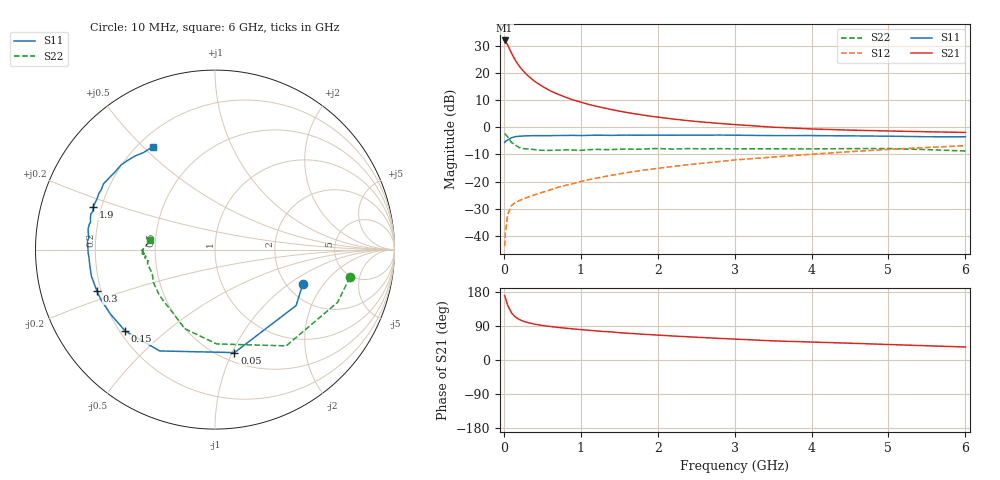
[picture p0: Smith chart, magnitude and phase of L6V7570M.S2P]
!  INFINEON TECHNOLOGIES Small Signal Semiconductors
! BFR380L3 , Si-NPN RF-Transistor in TSLP-3-1
!  Vce=0.75 V,  Ic=70 mA
! Common Emitter S-Parameters:  07. March 2005
#  GHz  S  MA  R  50
! f  S11  S21  S12  S22
! GHz  Mag  Ang  Mag  Ang  Mag  Ang  Mag  Ang
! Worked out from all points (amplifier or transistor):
!   36 points, 10 MHz to 6 GHz, reference 50 ohm
!   highest |S21| = 32.1 dB at 10 MHz (marker M1)
!   |S21| within 3 dB of that: start of sweep to 71.65 MHz
!   unconditionally stable (mu >= 1): 752.4 MHz to end of sweep
!   at 250 MHz: K = 0.60, MSG = 23.7 dB, |S12| = -26.4 dB
!   at 1.4 GHz: K = 1.11, MAG = 10.1 dB, |S12| = -17.7 dB
!   at 6 GHz: K = 1.04, MAG = 1.2 dB, |S12| = -6.8 dB
!   S11 on the Smith chart (normalised r, x): 10 MHz: 2.42, -1.30; 50 MHz: 0.59, -1.02; 150 MHz: 0.22, -0.37; 300 MHz: 0.18, -0.17; 1.9 GHz: 0.17, +0.17; 6 GHz: 0.26, +0.54
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0.01  0.5257 -21.7  40.24 170.2  0.0064 65.1  0.7671 -11.6
0.02  0.5491 -34.6  39.1 164.5  0.0113 69.1  0.7433 -23.3
0.05  0.584 -79.3  33.12 144.4  0.0247 56.1  0.6672 -53.5
0.1  0.6431 -118.6  23.39 124.2  0.036 44.5  0.5257 -89.0
0.15  0.6753 -137.8  17.24 113.3  0.0412 41.0  0.4717 -111.0
0.2  0.6842 -148.3  13.51 107.0  0.0444 41.3  0.424 -123.5
0.25  0.6933 -155.7  11.09 102.5  0.0476 41.1  0.4051 -135.2
0.3  0.6973 -160.5  9.319 99.3  0.0507 42.8  0.4004 -141.1
0.4  0.7043 -167.9  7.095 94.5  0.0567 46.3  0.3887 -152.1
0.5  0.7031 -172.7  5.722 91.2  0.0631 49.7  0.3765 -157.6
0.6  0.7032 -175.9  4.755 88.5  0.0699 52.4  0.3761 -161.2
0.7  0.7068 -178.5  4.111 86.1  0.0782 54.7  0.3796 -164.8
0.8  0.709 178.6  3.612 84.0  0.0847 57.1  0.3852 -167.2
0.9  0.7121 176.1  3.211 82.1  0.0914 58.5  0.3817 -169.6
1.1  0.7118 172.7  2.667 78.5  0.1078 60.4  0.3875 -171.0
1.5  0.7162 165.7  1.996 72.1  0.1381 62.2  0.3945 -174.4
1.9  0.7185 160.5  1.614 67.0  0.1681 62.7  0.4044 -176.3
2.2  0.7157 156.6  1.425 63.3  0.1899 62.4  0.3969 -177.1
3.5  0.7046 141.6  1.008 50.5  0.2832 59.4  0.4022 -179.2
4.5  0.6968 134.9  0.889 44.3  0.3557 56.4  0.4052 -179.6
5.5  0.6715 126.3  0.829 37.6  0.4252 51.2  0.3885 177.6
6  0.6702 121.1  0.807 34.3  0.4581 48.6  0.3656 171.9
